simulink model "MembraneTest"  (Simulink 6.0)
settings: Solver=ode45  StartTime=0.0  StopTime=SimTime  RelTol=1e-3
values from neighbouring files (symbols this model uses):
  b = S/Sm    (= 0.1)    [Constantes.m]    (also in ConstantesBck.m)
  C = 1    [Constantes.m]    (also in ConstantesBck.m)
  Fact = 10^2    (= 100)    [Constantes.m]    (also in ConstantesBck.m)
  gk = 36    [Constantes.m]    (also in ConstantesBck.m; sim_hh.m)
  gl = 0.3    [Constantes.m]    (also in ConstantesBck.m; sim_hh.m)
  gna = 120    [Constantes.m]    (also in ConstantesBck.m; sim_hh.m)
  h0 = 0.5961    [Constantes.m]    (also in ConstantesBck.m)
  IStim1 = AddI    (= 0)    [BiPhTest.m]    (also in ouin.m = -3000; TestStim.m; HalfSin.m; MonoAnoVSCath.m)
  IStim2 = -IStim1*i    [BiPhTest.m]    (also in ouin.m = 3000; TestStim.m = 0; MonoAnoVSCath.m = 0; MonoAnoVSCath_Prob.m = 0)
  m0 = 0.0529    [Constantes.m]    (also in ConstantesBck.m)
  mK = 0    [Constantes.m]    (also in ConstantesBck.m)
  mL = 0    [Constantes.m]    (also in ConstantesBck.m)
  mNa = 0    [Constantes.m]    (also in ConstantesBck.m)
  n0 = 0.3177    [Constantes.m]    (also in ConstantesBck.m)
  PerStim1 = TStim*(1+1/i)    [BiPhTest.m]    (also in ouin.m = 0.5; TestStim.m = i; MonoAnoVSCath.m = i*10; MonoAnoVSCath_Prob.m = i*10)
  PerStim2 = PerStim1    [BiPhTest.m]    (also in ouin.m = 0.5; TestStim.m; MonoAnoVSCath.m; MonoAnoVSCath_Prob.m)
  PhaseStim1 = 1    [BiPhTest.m]    (also in ouin.m; TestStim.m = 1+i; MonoAnoVSCath.m; MonoAnoVSCath_Prob.m)
  PhaseStim2 = PhaseStim1 + TStim    (= 6)    [BiPhTest.m]    (also in ouin.m = 1.25; TestStim.m = PhaseStim1 + PerStim2/2; MonoAnoVSCath.m = 1; MonoAnoVSCath_Prob.m = 1)
  Sm = 3.14e-2    (= 0.0314)    [Constantes.m]    (also in ConstantesBck.m = 0.000314)
  Vk = -82    [Constantes.m]    (also in ConstantesBck.m)
  Vl = -59    [Constantes.m]    (also in ConstantesBck.m)
  Vna = 45    [Constantes.m]    (also in ConstantesBck.m)
  Vr = -70    [Constantes.m]    (also in ConstantesBck.m)
  WidthStim1 = (1/(1+1/i))*100    [BiPhTest.m]    (also in ouin.m = 50; TestStim.m = 50; MonoAnoVSCath.m = 5; MonoAnoVSCath_Prob.m = 5)
  WidthStim2 = (1/(1+i))*100    [BiPhTest.m]    (also in ouin.m = 50; TestStim.m = 50; MonoAnoVSCath.m = 5; MonoAnoVSCath_Prob.m = 5)

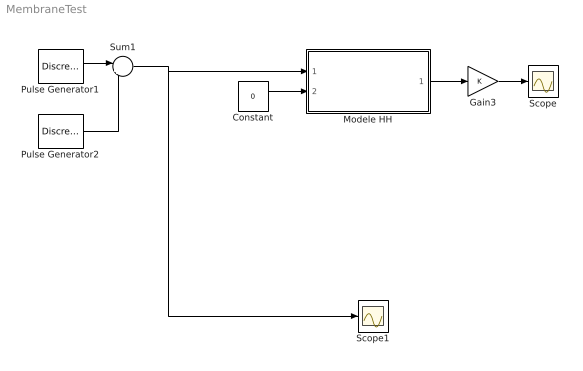
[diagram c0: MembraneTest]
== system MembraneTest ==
  Constant : Constant  Value=0
  Gain3 : Gain
  Modele HH : Subsystem
  Pulse Generator1 : DiscretePulseGenerator  PulseType=Time based  Amplitude=IStim1  Period=PerStim1  PulseWidth=WidthStim1  PhaseDelay=PhaseStim1
  Pulse Generator2 : DiscretePulseGenerator  PulseType=Time based  Amplitude=IStim2  Period=PerStim2  PulseWidth=WidthStim2  PhaseDelay=PhaseStim2
  Scope : Scope
  Scope1 : Scope
  Sum1 : Sum  Inputs=|++
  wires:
  Modele HH/1(HHout) -> Gain3/1
  Constant/1 -> Modele HH/2(VRefIn)
  Pulse Generator1/1 -> Sum1/1
  Gain3/1 -> Scope/1
  Sum1/1 -> Modele HH/1(HHin), Scope1/1
  Pulse Generator2/1 -> Sum1/2

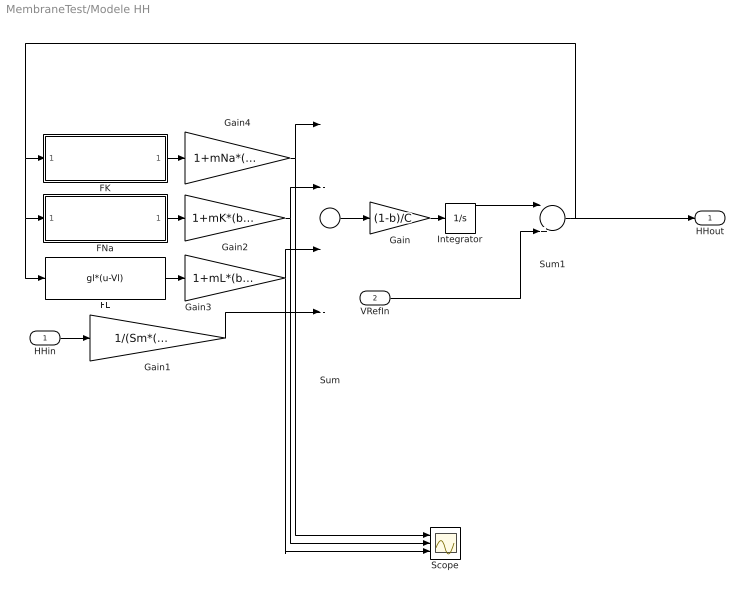
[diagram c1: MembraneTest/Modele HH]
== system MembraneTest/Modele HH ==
  HHin : Inport  Port=1  LatchInput=off
  VRefIn : Inport  Port=2  LatchInput=off
  FK : Subsystem
  FL : Fcn  Expr=gl*(u-Vl)
  FNa : Subsystem
  Gain : Gain  Gain=(1-b)/C
  Gain1 : Gain  Gain=1/(Sm*(1-b)*Fact)
  Gain2 : Gain  Gain=1+mK*(b/(1-b))
  Gain3 : Gain  Gain=1+mL*(b/(1-b))
  Gain4 : Gain  Gain=1+mNa*(b/(1-b))
  Integrator : Integrator  InitialCondition=Vr
  Scope : Scope  NumInputPorts=3
  Sum : Sum  Inputs=|---+
  Sum1 : Sum  Inputs=|++
  HHout : Outport
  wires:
  Sum/1 -> Gain/1
  Gain/1 -> Integrator/1
  FK/1(FKout) -> Gain4/1
  FNa/1(FNaOut) -> Gain2/1
  FL/1 -> Gain3/1
  HHin/1 -> Gain1/1
  Integrator/1 -> Sum1/1
  Sum1/1 -> FNa/1(FNaIn), FL/1, FK/1(FKIn), HHout/1
  Gain1/1 -> Sum/4
  Gain4/1 -> Sum/1, Scope/1
  Gain2/1 -> Sum/2, Scope/2
  Gain3/1 -> Sum/3, Scope/3
  VRefIn/1 -> Sum1/2

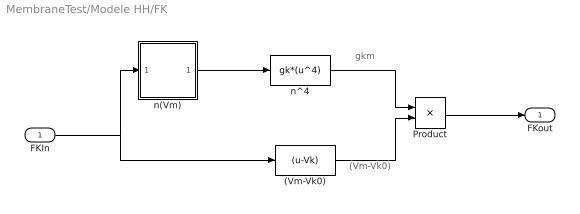
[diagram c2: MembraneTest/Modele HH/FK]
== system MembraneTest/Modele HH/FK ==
  note: gkm
  note: (Vm-Vk0)
  FKIn : Inport  Port=1  LatchInput=off
  (Vm-Vk0) : Fcn  Expr=(u-Vk)
  Product : Product
  n(Vm) : Subsystem
  n^4 : Fcn  Expr=gk*(u^4)
  FKout : Outport  InitialOutput=0
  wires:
  n(Vm)/1(n) -> n^4/1
  (Vm-Vk0)/1 -> Product/2
  Product/1 -> FKout/1
  n^4/1 -> Product/1
  FKIn/1 -> n(Vm)/1(Vm), (Vm-Vk0)/1

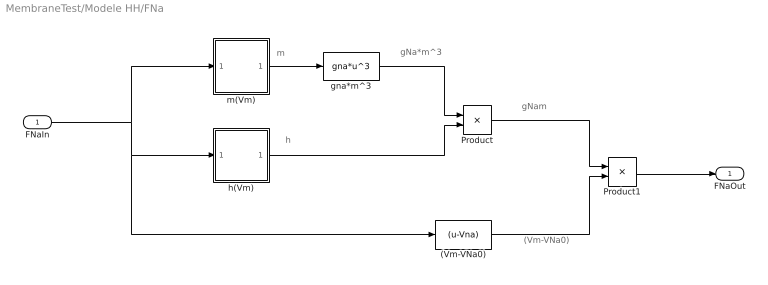
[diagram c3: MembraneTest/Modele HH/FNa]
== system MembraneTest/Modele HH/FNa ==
  note: gNa*m^3
  note: m
  note: h
  note: gNam
  note: (Vm-VNa0)
  FNaIn : Inport  Port=1  LatchInput=off
  (Vm-VNa0) : Fcn  Expr=(u-Vna)
  Product : Product
  Product1 : Product
  gna*m^3 : Fcn  Expr=gna*u^3
  h(Vm) : Subsystem
  m(Vm) : Subsystem
  FNaOut : Outport  InitialOutput=0
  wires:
  (Vm-VNa0)/1 -> Product1/2
  gna*m^3/1 -> Product/1
  Product1/1 -> FNaOut/1
  FNaIn/1 -> m(Vm)/1(Vm), h(Vm)/1(Vm), (Vm-VNa0)/1
  m(Vm)/1(n) -> gna*m^3/1
  h(Vm)/1(h) -> Product/2
  Product/1 -> Product1/1

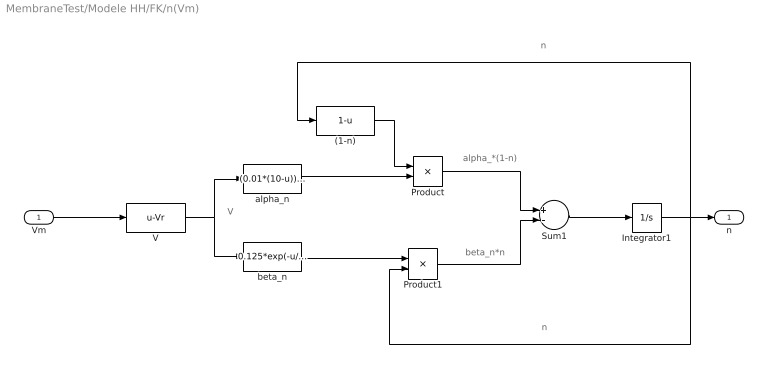
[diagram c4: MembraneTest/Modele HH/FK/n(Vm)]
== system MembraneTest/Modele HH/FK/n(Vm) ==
  note: V
  note: alpha_*(1-n)
  note: beta_n*n
  note: n
  note: n
  Vm : Inport  Port=1  LatchInput=off
  (1-n) : Fcn  Expr=1-u
  Integrator1 : Integrator  InitialCondition=n0
  Product : Product
  Product1 : Product
  Sum1 : Sum  Inputs=+-
  V : Fcn  Expr=u-Vr
  alpha_n : Fcn  Expr=(0.01*(10-u))/(exp((10-u)/10)-1)
  beta_n : Fcn  Expr=0.125*exp(-u/80)
  n : Outport  InitialOutput=0
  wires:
  V/1 -> alpha_n/1, beta_n/1
  alpha_n/1 -> Product/2
  (1-n)/1 -> Product/1
  beta_n/1 -> Product1/1
  Product/1 -> Sum1/1
  Product1/1 -> Sum1/2
  Sum1/1 -> Integrator1/1
  Integrator1/1 -> (1-n)/1, Product1/2, n/1
  Vm/1 -> V/1

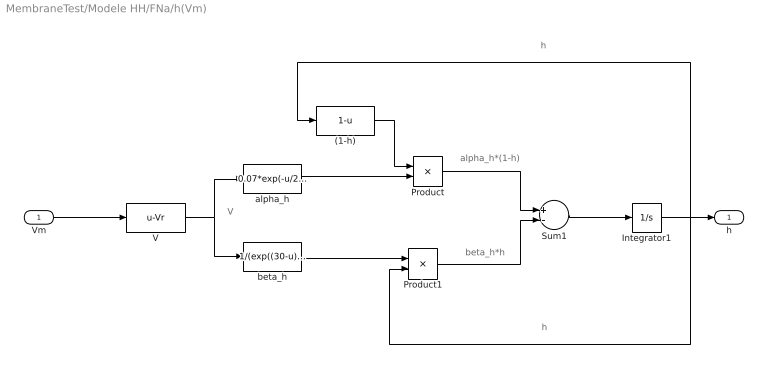
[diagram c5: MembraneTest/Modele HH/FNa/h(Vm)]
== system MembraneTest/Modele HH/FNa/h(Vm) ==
  note: h
  note: h
  note: beta_h*h
  note: alpha_h*(1-h)
  note: V
  Vm : Inport  Port=1  LatchInput=off
  (1-h) : Fcn  Expr=1-u
  Integrator1 : Integrator  InitialCondition=h0
  Product : Product
  Product1 : Product
  Sum1 : Sum  Inputs=+-
  V : Fcn  Expr=u-Vr
  alpha_h : Fcn  Expr=0.07*exp(-u/20)
  beta_h : Fcn  Expr=1/(exp((30-u)/10)+1)
  h : Outport  InitialOutput=0
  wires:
  Vm/1 -> V/1
  Integrator1/1 -> h/1, Product1/2, (1-h)/1
  Sum1/1 -> Integrator1/1
  Product1/1 -> Sum1/2
  Product/1 -> Sum1/1
  beta_h/1 -> Product1/1
  (1-h)/1 -> Product/1
  alpha_h/1 -> Product/2
  V/1 -> beta_h/1, alpha_h/1

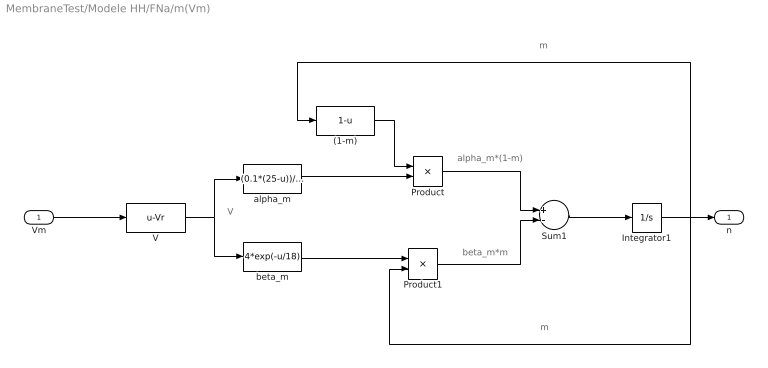
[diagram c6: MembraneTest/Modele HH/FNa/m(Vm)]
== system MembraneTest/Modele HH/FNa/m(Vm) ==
  note: m
  note: m
  note: beta_m*m
  note: alpha_m*(1-m)
  note: V
  Vm : Inport  Port=1  LatchInput=off
  (1-m) : Fcn  Expr=1-u
  Integrator1 : Integrator  InitialCondition=m0
  Product : Product
  Product1 : Product
  Sum1 : Sum  Inputs=+-
  V : Fcn  Expr=u-Vr
  alpha_m : Fcn  Expr=(0.1*(25-u))/(exp((25-u)/10)-1)
  beta_m : Fcn  Expr=4*exp(-u/18)
  n : Outport  InitialOutput=0
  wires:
  Vm/1 -> V/1
  Integrator1/1 -> n/1, Product1/2, (1-m)/1
  Sum1/1 -> Integrator1/1
  Product1/1 -> Sum1/2
  Product/1 -> Sum1/1
  beta_m/1 -> Product1/1
  (1-m)/1 -> Product/1
  alpha_m/1 -> Product/2
  V/1 -> beta_m/1, alpha_m/1
